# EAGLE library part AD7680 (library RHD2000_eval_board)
Analog Devices AD7680 16-bit ADC
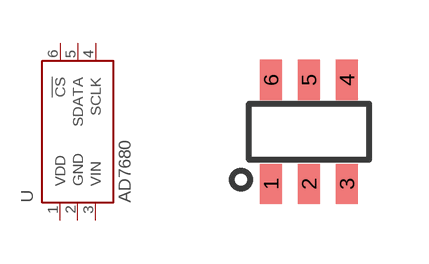
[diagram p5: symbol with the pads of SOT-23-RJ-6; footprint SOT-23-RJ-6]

Designator prefix U

## AD7680-SOT-23  [SOT-23-RJ-6]
1  VDD  pwr
2  GND  pwr
3  VIN  in
4  SCLK  in
5  SDATA  out
6  !CS!  in

## Footprint SOT-23-RJ-6 (pad centres in mm)
smd 0.55 x 1: 1 -0.95,-1.3; 2 0,-1.3; 3 0.95,-1.3; 4 0.95,1.3; 5 0,1.3; 6 -0.95,1.3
